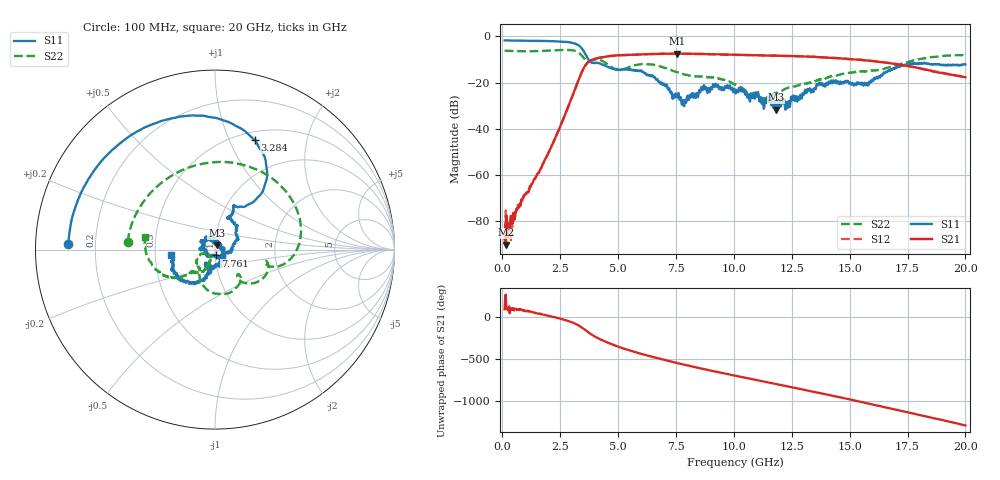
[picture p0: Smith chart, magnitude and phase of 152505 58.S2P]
!  2-Port S-parameters saved by WinCal
! VAR MeasName=S-Parameters (CALIBRATED_DATA) read from VNA (N5230C)
! VAR MeasDate=4/10/2015 9:34:38 AM
! VAR NAME=152505 58
! VAR FILENAME=152505 58.S2P
! VAR DATE=4/10/2015 9:34:38 AM
! VAR PHYS_PORTS=1,2
# Hz S DB R 50
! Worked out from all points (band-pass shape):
!   801 points, 100 MHz to 20 GHz, reference 50 ohm
!   highest |S21| = -7.45 dB at 7.538 GHz (marker M1); lowest = -90.3 dB at 149.8 MHz (marker M2)
!   |S21| within 3 dB of the highest: 3.807 GHz to 15.76 GHz (11.95 GHz wide, 122 % of centre)
!   lowest |S11| = -31.8 dB at 11.82 GHz (marker M3), VSWR 1.05, Z = 50.9 + j2.43 ohm
!   |S11| at or under -10 dB: 3.716 GHz to end of sweep
!   |S22| runs from -27.0 to -5.8 dB; largest |S21 - S12| = 0.0052
!   S11 on the Smith chart (normalised r, x): 100 MHz: 0.10, +0.02; 3.284 GHz: 0.60, +1.25; 7.761 GHz: 1.00, -0.07; 20 GHz: 0.60, -0.04
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1e8  -1.75 177.6  -87.97 95.0  -89.46 39.5  -6.23 174.9
1.4975e8  -1.75 176.5  -90.27 -88.6  -75.43 77.7  -6.23 172.3
4.4825e8  -1.77 169.3  -81.18 95.8  -81.81 99.7  -6.31 157.3
1.965625e9  -2.01 130.0  -51.05 19.2  -51.00 18.4  -6.17 83.4
3.284e9  -3.77 69.9  -19.01 -95.8  -19.05 -95.9  -6.94 -1.7
3.43325e9  -5.19 58.8  -15.41 -121.8  -15.44 -121.8  -8.26 -12.6
3.806375e9  -11.01 58.1  -10.45 162.8  -10.48 162.6  -10.73 -12.4
4.303875e9  -12.09 65.1  -9.02 87.6  -9.03 87.5  -10.53 -37.0
5.1745e9  -14.20 67.9  -8.08 -6.8  -8.13 -6.8  -14.38 -45.9
5.945625e9  -14.93 46.3  -7.83 -72.1  -7.84 -71.8  -12.08 -65.5
6.741625e9  -19.73 15.7  -7.55 -130.7  -7.57 -130.9  -12.79 -100.4
7.537625e9  -26.43 -52.4  -7.45 175.1  -7.47 175.2  -15.53 -121.4
7.7615e9  -29.64 -84.9  -7.47 160.2  -7.48 160.5  -16.20 -124.8
8.831125e9  -23.02 -180.0  -7.65 93.7  -7.71 93.7  -17.68 -136.5
1.005e10  -23.37 122.6  -7.94 22.9  -7.97 22.9  -20.98 -159.4
1.109475e10  -28.14 103.6  -8.20 -36.0  -8.18 -36.2  -26.74 -141.4
1.181612e10  -31.80 68.0  -8.33 -76.4  -8.36 -76.7  -24.49 -115.8
1.338325e10  -23.00 -51.9  -8.84 -165.8  -8.81 -165.5  -19.65 -113.7
1.500012e10  -20.03 -119.3  -9.79 99.6  -9.83 99.9  -15.72 -129.1
1.669162e10  -14.62 -109.6  -11.53 -2.8  -11.50 -3.2  -13.46 -136.9
1.796025e10  -12.03 -148.4  -13.62 -82.9  -13.72 -82.4  -9.87 -152.8
2e10  -12.13 -173.6  -17.68 148.7  -17.67 149.0  -8.09 170.0
